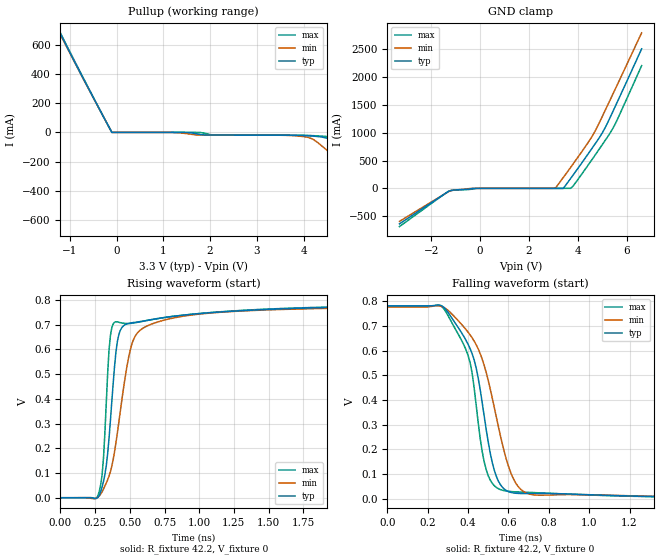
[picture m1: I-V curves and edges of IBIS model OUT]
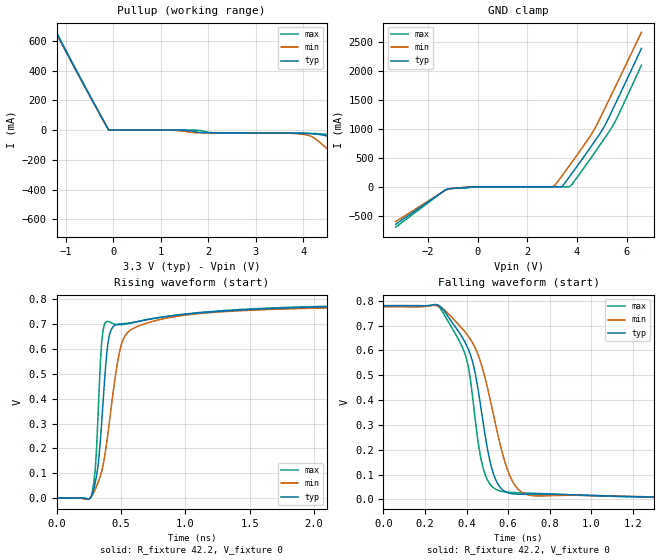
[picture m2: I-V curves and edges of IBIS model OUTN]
|   IBIS File of SG2520HHN C
|   HCSL Zdiff=85, Vcc=3.3V, fo>212.5MHz
[IBIS Ver]   3.2
[File Name]   sg2520hhn_hf_85_33v.ibs
[File Rev]   1.0
[Date]   Aug. 4, 2020
[Source]
[Notes]
Created by Minoru Kozaki
[Disclaimer]
Seiko Epson Corporation makes no warranty with respect to the
information contained herein.
[Copyright]
Copyright(C) 2020, Seiko Epson Corporation. All rights reserved.
|   Component
[Component]   SG2520HHN
[Manufacturer]  Seiko Epson Corporation
[Package]
R_pkg   17.7m   NA   NA
L_pkg   235p   NA   NA
C_pkg   208f   NA   NA
[Pin]   signal_name   model_name   R_pin   L_pin   C_pin
1   OE/ST   NC
2   NC   NC
3   GND   GND
4   OUT   OUT   17.7m   235p   208f
5   OUTN   OUTN   10.4m   129p   221f
6   VCC   POWER
[Diff Pin] inv_pin  vdiff  tdelay_typ
4   5   0   0
| Models and submodels in the file (2): OUT (Open_source), OUTN (Open_source)
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|   Model OUT
[Model]   OUT
Model_type   Open_source
Polarity   Non-Inverting
Vref = 0
Vmeas = 0.4
Rref = 42.2
Cref = 0
C_comp   12.0p   12.0p   12.0p
[Temperature Range]   25   105   -40
[Voltage Range]   3.3   2.97   3.63
[Pullup Reference]   3.3   2.97   3.63
[GND Clamp Reference]   0   0   0
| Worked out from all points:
|   GND clamp passes 1 mA (typ) near -0.23 V on its own axis
|   falling waveform, R_fixture 42.2, V_fixture 0: 20-80 % time 117ps typ, 150ps min, 100ps max; typ from 0.781 V to 0 V
|   rising waveform, R_fixture 42.2, V_fixture 0: 20-80 % time 72.6ps typ, 134ps min, 45.1ps max; typ from 0 V to 0.78 V
[Pullup]
-3.3V     2.511A     2.489A     2.536A
-1.3V     738.7mA    733.7mA    747.4mA
-1.2V     675.4mA    670.8mA    683.1mA
-100mV    32.53uA    19.73uA    91.96uA
1.7V      -8.637mA   -17.25mA   -82.98uA
2.1V      -18.17mA   -18.36mA   -17.38mA
3.9V      -20.86mA   -25.48mA   -19.14mA
4.2V      -25.41mA   -46.3mA    -22.26mA
4.5V      -39.69mA   -122mA     -28.13mA
4.8V      -114.5mA   -202.1mA   -39.68mA
5V        -172.9mA   -255.5mA   -76.13mA
6.6V      -641.1mA   -684.5mA   -583.3mA
[GND Clamp]
-3.3V     -639.8mA   -594.8mA   -688.3mA
-1.4V     -84.3mA    -86.81mA   -84.01mA
-1.2V     -38.8mA    -41.15mA   -40.33mA
-100mV    -30.13uA   -16uA      -185.9uA
3.1V      -1.477uA   17.81mA    -3.234uA
3.4V      32.53uA    197.2mA    -2.45uA
3.7V      179.9mA    378.5mA    30.98uA
3.8V      240.6mA    440.1mA    41.86mA
4.6V      738.7mA    954.1mA    535.9mA
5V        1.004A     1.302A     792.5mA
5.5V      1.455A     1.767A     1.142A
6.6V      2.511A     2.8A       2.209A
[Falling Waveform]
R_fixture = 42.2
V_fixture = 0
V_fixture_min = 0
V_fixture_max = 0
0s        780.7mV    776.1mV    780.6mV
260ps     783.8mV    780.3mV    782mV
350ps     694.4mV    721.8mV    667.8mV
410ps     607.9mV    663.4mV    551.2mV
450ps     489.6mV    607mV      309.6mV
490ps     280mV      510.5mV    117.2mV
540ps     90.77mV    331mV      45.84mV
610ps     26.06mV    109mV      29.27mV
740ps     21.75mV    14.69mV    24.4mV
4ns       189uV      248uV      180uV
[Rising Waveform]
R_fixture = 42.2
V_fixture = 0
V_fixture_min = 0
V_fixture_max = 0
0s        78uV       94uV       84uV
280ps     10.27mV    7.35mV     25.33mV
310ps     65.76mV    35.08mV    158.9mV
350ps     240.3mV    87.46mV    596.5mV
370ps     388.2mV    127.6mV    687.7mV
390ps     532.1mV    186.7mV    709.9mV
430ps     675.5mV    343.9mV    708.7mV
520ps     708.3mV    630.5mV    706.3mV
720ps     726.9mV    714.3mV    726.4mV
4ns       780mV      775.1mV    780.1mV
[Ramp]
R_load = 42.2
dV/dt_r   0.47040/72.78p   0.46656/134.73p   0.47105/44.91p
dV/dt_f   0.47040/118.19p   0.46656/150.05p   0.47105/101.82p
|   Model OUTN
[Model]   OUTN
Model_type   Open_source
Polarity   Inverting
Vref = 0
Vmeas = 0.4
Rref = 42.2
Cref = 0
C_comp   12.0p   12.0p   12.0p
[Temperature Range]   25   105   -40
[Voltage Range]   3.3   2.97   3.63
[Pullup Reference]   3.3   2.97   3.63
[GND Clamp Reference]   0   0   0
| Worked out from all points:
|   GND clamp passes 1 mA (typ) near -0.23 V on its own axis
|   falling waveform, R_fixture 42.2, V_fixture 0: 20-80 % time 115ps typ, 148ps min, 97.7ps max; typ from 0.78 V to 0 V
|   rising waveform, R_fixture 42.2, V_fixture 0: 20-80 % time 72ps typ, 135ps min, 44.4ps max; typ from 0 V to 0.779 V
[Pullup]
-3.3V     2.386A     2.369A     2.406A
-1.3V     712.9mA    708.1mA    721.2mA
-1.2V     651.8mA    647.5mA    659.1mA
-100mV    32.53uA    19.73uA    91.97uA
1.7V      -8.61mA    -17.23mA   -82.97uA
2.1V      -18.16mA   -18.35mA   -17.37mA
3.9V      -20.85mA   -25.47mA   -19.14mA
4.2V      -25.4mA    -46.31mA   -22.25mA
4.5V      -39.68mA   -122.8mA   -28.12mA
4.8V      -115.3mA   -203.7mA   -39.69mA
5V        -174.4mA   -257.7mA   -76.6mA
6.6V      -648mA     -691.2mA   -590.1mA
[GND Clamp]
-3.3V     -646.7mA   -600.5mA   -696.4mA
-1.4V     -84.81mA   -87.25mA   -84.64mA
-1.2V     -38.8mA    -41.14mA   -40.36mA
-100mV    -30.13uA   -16uA      -185.8uA
3.1V      -1.477uA   17.19mA    -3.234uA
3.4V      32.53uA    190.3mA    -2.451uA
3.7V      173.6mA    365.3mA    30.98uA
4.3V      529.7mA    726.4mA    336.1mA
4.7V      774.2mA    989.7mA    578.6mA
5V        965.2mA    1.241A     764.7mA
5.5V      1.385A     1.683A     1.093A
6.6V      2.386A     2.663A     2.097A
[Falling Waveform]
R_fixture = 42.2
V_fixture = 0
V_fixture_min = 0
V_fixture_max = 0
0s        780.1mV    775.4mV    779.9mV
260ps     783.4mV    779.1mV    780.3mV
360ps     677.3mV    705.3mV    645.8mV
400ps     620mV      666.4mV    564.8mV
430ps     550.5mV    628.4mV    404.8mV
490ps     253.5mV    485.9mV    97.97mV
540ps     78.89mV    299.2mV    40.82mV
610ps     24.03mV    91.06mV    28.23mV
740ps     21.5mV     13.93mV    23.94mV
4ns       185uV      242uV      177uV
[Rising Waveform]
R_fixture = 42.2
V_fixture = 0
V_fixture_min = 0
V_fixture_max = 0
0s        74uV       99uV       83uV
270ps     6.271mV    6.122mV    9.933mV
300ps     60.78mV    34.76mV    111.2mV
330ps     168.1mV    73.44mV    425.5mV
350ps     299.6mV    106.4mV    623mV
390ps     581.7mV    224.1mV    711mV
430ps     683.7mV    386.8mV    704.6mV
510ps     701.9mV    628.5mV    698.3mV
730ps     720.8mV    708.9mV    721.2mV
4ns       779.3mV    774.3mV    779.4mV
[Ramp]
R_load = 42.2
dV/dt_r   0.47036/72.50p   0.46652/136.06p   0.47098/44.40p
dV/dt_f   0.47036/115.96p   0.46652/148.29p   0.47098/99.47p
